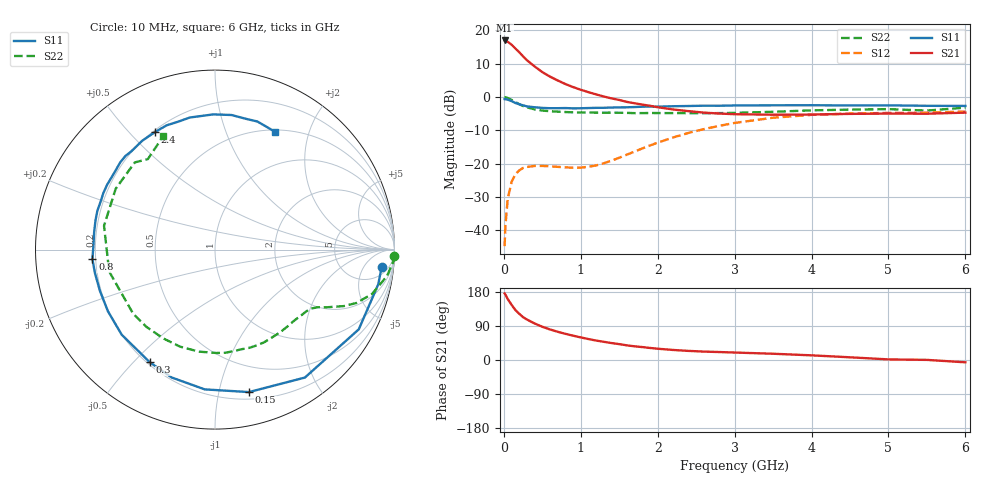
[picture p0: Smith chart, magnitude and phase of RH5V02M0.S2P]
! SIEMENS Small Signal Semiconductors
! BFR106
! Si NPN RF Bipolar Junction Transistor in SOT23
! VCE = 5 V  IC = 2 mA
! Common Emitter S-Parameters:  August  1996
# GHz  S  MA  R  50
!  f  S11  S21  S12  S22
! GHz  MAG  ANG  MAG  ANG  MAG  ANG  MAG  ANG
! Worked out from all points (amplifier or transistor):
!   36 points, 10 MHz to 6 GHz, reference 50 ohm
!   highest |S21| = 17.0 dB at 10 MHz (marker M1)
!   |S21| within 3 dB of that: start of sweep to 176.4 MHz
!   unconditionally stable (mu >= 1): 792.8 MHz to 1.841 GHz; 4.018 GHz to end of sweep
!   at 250 MHz: K = 0.32, MSG = 16.7 dB, |S12| = -21.3 dB
!   at 1.4 GHz: K = 1.25, MAG = 6.3 dB, |S12| = -19.1 dB
!   at 6 GHz: K = 1.02, MAG = -1.0 dB, |S12| = -4.3 dB
!   S11 on the Smith chart (normalised r, x): 10 MHz: 9, -13; 150 MHz: 0.26, -1.23; 300 MHz: 0.21, -0.56; 800 MHz: 0.19, -0.04; 2.4 GHz: 0.21, +0.59; 6 GHz: 0.52, +1.50
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0.01  0.9337 -6.0  7.077 175.5  0.0058 89.2  0.998 -1.9
0.02  0.9299 -12.0  7.006 172.7  0.0115 83.7  0.9963 -3.7
0.05  0.916 -29.0  6.759 161.1  0.0295 74.3  0.97 -8.7
0.1  0.8713 -54.9  6.133 145.9  0.0532 61.0  0.909 -15.8
0.15  0.816 -76.6  5.364 131.9  0.0695 50.3  0.8417 -20.7
0.2  0.7809 -94.2  4.714 122.0  0.0795 42.9  0.7832 -23.7
0.25  0.7523 -108.7  4.088 113.1  0.0864 37.3  0.7342 -25.7
0.3  0.7254 -120.0  3.583 106.8  0.0895 33.7  0.7027 -27.2
0.4  0.7036 -137.6  2.884 96.4  0.0926 28.7  0.6543 -29.4
0.5  0.6884 -150.1  2.371 87.7  0.0928 26.7  0.6275 -31.6
0.6  0.6811 -160.3  2.03 80.6  0.0916 26.6  0.6141 -34.1
0.8  0.685 -175.6  1.57 69.1  0.0883 31.0  0.5966 -40.0
1.1  0.6853 166.3  1.185 55.3  0.0902 46.1  0.5865 -50.5
1.6  0.7032 144.7  0.847 38.6  0.1369 68.4  0.5799 -70.6
2.2  0.7295 123.8  0.652 26.5  0.2479 69.4  0.5754 -98.9
2.4  0.7351 117.2  0.616 24.0  0.29 66.4  0.5747 -109.8
3.5  0.7534 90.7  0.544 16.5  0.4905 41.2  0.6021 -168.3
4  0.7555 83.0  0.548 12.3  0.5414 29.3  0.6323 167.9
4.5  0.7487 76.6  0.56 7.1  0.5666 18.7  0.6489 148.5
5  0.7518 71.7  0.566 1.6  0.5788 10.1  0.6601 132.6
5.5  0.7405 66.3  0.563 0.3  0.5827 6.0  0.6278 126.6
6  0.7365 63.2  0.585 -6.1  0.6082 -2.1  0.6946 114.5
